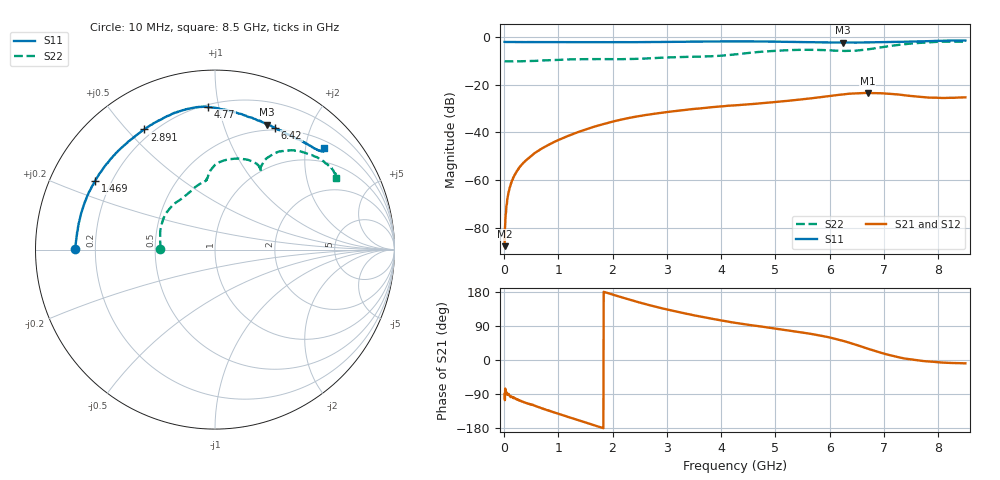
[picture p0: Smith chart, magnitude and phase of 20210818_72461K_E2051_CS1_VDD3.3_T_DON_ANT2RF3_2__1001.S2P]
!Agilent Technologies,E5071C,MY46417908,A.11.23
!Date: Wed Aug 18 14:30:25 2021
!Data & Calibration Information:
!Freq	S11:SOLT2(ON)	S21:SOLT2(ON)	S12:SOLT2(ON)	S22:SOLT2(ON)
!PortZ  Port1:50+j0  Port2:50+j0
!Above PortZ is port z conversion or system Z0 setting when saving the data.
!When reading, reference impedance value at option line is always used.
# Hz S dB R 50
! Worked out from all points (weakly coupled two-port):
!   1601 points, 10 MHz to 8.5 GHz, reference 50 ohm
!   highest |S21| = -23.49 dB at 6.701 GHz (marker M1); lowest = -87.5 dB at 10 MHz (marker M2)
!   lowest |S11| = -2.5 dB at 6.25 GHz (marker M3), VSWR 7.13, Z = 21.9 + j70.5 ohm
!   |S11| at or under -10 dB: nowhere
!   |S22| runs from -10.3 to -2.0 dB; largest |S21 - S12| = 0.00035
!   S11 on the Smith chart (normalised r, x): 10 MHz: 0.12, +0.00; 1.469 GHz: 0.14, +0.26; 2.891 GHz: 0.17, +0.56; 4.77 GHz: 0.22, +0.93; 6.42 GHz: 0.48, +1.50; 8.5 GHz: 0.65, +2.39
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1e7  -2.15 179.7  -87.48 -89.7  -82.90 -84.7  -10.28 179.6
7.3675e7  -2.19 178.4  -66.06 -89.4  -66.45 -91.2  -10.29 178.2
1.214312e8  -2.20 177.4  -61.75 -98.0  -61.64 -97.0  -10.30 177.1
2.063312e8  -2.22 175.7  -57.25 -101.7  -57.18 -102.8  -10.30 175.2
3.124562e8  -2.23 173.4  -53.80 -108.8  -53.74 -108.1  -10.25 173.0
5.247062e8  -2.23 169.2  -49.35 -118.7  -49.34 -118.5  -10.12 168.6
7.210375e8  -2.24 165.0  -46.36 -128.5  -46.37 -128.9  -9.92 163.4
1.426769e9  -2.27 151.0  -39.31 -161.5  -39.34 -161.6  -9.38 142.0
1.469219e9  -2.28 150.1  -39.00 -163.4  -39.01 -163.3  -9.38 140.7
2.17495e9  -2.27 135.5  -34.53 165.0  -34.53 165.1  -9.37 121.9
2.843538e9  -2.20 121.3  -31.94 138.6  -31.93 138.5  -8.84 108.8
2.891294e9  -2.20 120.4  -31.80 137.1  -31.80 137.0  -8.78 108.0
4.255e9  -1.95 98.7  -28.66 98.2  -28.65 98.2  -7.39 94.4
4.769706e9  -1.99 92.7  -27.72 87.7  -27.72 87.8  -6.22 86.9
5.671769e9  -2.29 78.9  -25.69 68.5  -25.71 68.6  -5.48 65.7
6.25015e9  -2.45 67.3  -24.09 50.3  -24.12 50.2  -5.94 59.8
6.41995e9  -2.43 63.7  -23.74 42.9  -23.75 42.7  -5.87 60.0
6.701181e9  -2.40 57.7  -23.49 29.8  -23.52 29.7  -5.30 61.0
7.088538e9  -2.21 51.2  -23.83 13.5  -23.85 13.3  -3.95 58.0
7.497119e9  -2.06 45.7  -24.75 1.5  -24.75 1.4  -2.86 49.8
8.006519e9  -1.73 42.1  -25.52 -6.2  -25.50 -6.2  -2.12 37.6
8.5e9  -1.61 43.0  -25.35 -8.7  -25.32 -8.9  -2.13 30.8
